FUNCTION_BLOCK FB_IEDServerSession IMPLEMENTS I_ScsmAbortIndEventSink, I_ScsmAssociateIndEventSink, I_ScsmReleaseIndEventSink
VAR_INPUT
	fbConnection		: FB_iec61850ConnectionClass := (ipAbortInd:=THIS^, ipAssociateInd:=THIS^, ipReleaseInd:=THIS^);
END_VAR
VAR
	_bAbort				: BOOL; (* Rising edge activates AbortReq() command execution *)
	_bDisconnect		: BOOL; (* Rising edge activates ReleaseReq() command execution *)
	
	state				: BYTE;
	eState				: E_AsyncEnvironmentState; (* Environment state *)
	bBusy				: BOOL; (* If TRUE => command execution is busy *)
	bSuccess			: BOOL;
	ipResult			: I_AsyncServiceResultClass;
	sLastErrorResult	: T_MaxString;
	fbAbortReason		: FB_ServiceErrorClass := (stError:=SUCCESS_EVENT);
	sLastAbortReason	: T_MaxString;
END_VAR

fbConnection.Execute();
eState:= fbConnection.eState;

(* Execute server control block implementations *)
fbIED.IEDLD1.LLN0.urcb101.Server.Execute();
fbIED.IEDLD1.LLN0.brcb101.Server.Execute();

{region Controlmodel}
fbIED.IEDLD1.ATCC1.BndCtrChg.fbControl.Execute();
fbIED.IEDLD1.ATCC1.TapChg.fbControl.Execute();
fbIED.IEDLD1.ATCC1.TapPos.fbControl.Execute();

fbIED.IEDLD1.CSWI1.Pos.fbControl.Execute();

fbIED.IEDLD1.LEDGGIO1.AnOut1.fbControl.Execute();
fbIED.IEDLD1.LEDGGIO1.DPCSO1.fbControl.Execute();
fbIED.IEDLD1.LEDGGIO1.ISCSO1.fbControl.Execute();
fbIED.IEDLD1.LEDGGIO1.SPCSO1.fbControl.Execute();

fbIED.IEDLD1.LEDGGIO2.AnOut1.fbControl.Execute();
fbIED.IEDLD1.LEDGGIO2.DPCSO1.fbControl.Execute();
fbIED.IEDLD1.LEDGGIO2.ISCSO1.fbControl.Execute();
fbIED.IEDLD1.LEDGGIO2.SPCSO1.fbControl.Execute();

fbIED.IEDLD1.LEDGGIO3.AnOut1.fbControl.Execute();
fbIED.IEDLD1.LEDGGIO3.DPCSO1.fbControl.Execute();
fbIED.IEDLD1.LEDGGIO3.ISCSO1.fbControl.Execute();
fbIED.IEDLD1.LEDGGIO3.SPCSO1.fbControl.Execute();

fbIED.IEDLD1.LEDGGIO4.AnOut1.fbControl.Execute();
fbIED.IEDLD1.LEDGGIO4.DPCSO1.fbControl.Execute();
fbIED.IEDLD1.LEDGGIO4.ISCSO1.fbControl.Execute();
fbIED.IEDLD1.LEDGGIO4.SPCSO1.fbControl.Execute();

fbIED.IEDLD1.LEDGGIO5.AnOut1.fbControl.Execute();
fbIED.IEDLD1.LEDGGIO5.DPCSO1.fbControl.Execute();
fbIED.IEDLD1.LEDGGIO5.ISCSO1.fbControl.Execute();
fbIED.IEDLD1.LEDGGIO5.SPCSO1.fbControl.Execute();

fbIED.IEDLD1.LEDGGIO6.AnOut1.fbControl.Execute();
fbIED.IEDLD1.LEDGGIO6.DPCSO1.fbControl.Execute();
fbIED.IEDLD1.LEDGGIO6.ISCSO1.fbControl.Execute();
fbIED.IEDLD1.LEDGGIO6.SPCSO1.fbControl.Execute();

fbIED.IEDLD1.LEDGGIO7.AnOut1.fbControl.Execute();
fbIED.IEDLD1.LEDGGIO7.DPCSO1.fbControl.Execute();
fbIED.IEDLD1.LEDGGIO7.ISCSO1.fbControl.Execute();
fbIED.IEDLD1.LEDGGIO7.SPCSO1.fbControl.Execute();

fbIED.IEDLD1.LEDGGIO8.AnOut1.fbControl.Execute();
fbIED.IEDLD1.LEDGGIO8.DPCSO1.fbControl.Execute();
fbIED.IEDLD1.LEDGGIO8.ISCSO1.fbControl.Execute();
fbIED.IEDLD1.LEDGGIO8.SPCSO1.fbControl.Execute();

fbIED.IEDLD1.XCBR1.Pos.fbControl.Execute();

fbIED.IEDLD1.LLN0.Mod_.fbControl.Execute();
{endregion}

CASE state OF
	0: (* Initial state *)
		IF _bAbort THEN (* Abort connection => execute AbortReq() command *)
			_bAbort:= FALSE;
			bSuccess:= fbConnection.AbortReq(ipReason:=fbAbortReason, ipSink:=0, ipResult=>ipResult);
			state:= SEL(bSuccess, 100, 1);
		ELSIF eState = E_AsyncEnvironmentState.Established AND _bDisconnect THEN (* Close/release connection => execute ReleaseReq() command *)
			_bDisconnect:= FALSE;
			bSuccess:= fbConnection.ReleaseReq(ipSink:=0, ipResult=>ipResult);
			state:= SEL(bSuccess, 100, 1);
		ELSIF eState = E_AsyncEnvironmentState.Established THEN (* Connection established => exchange IED data *)
			state:= 10;
		END_IF
		_bDisconnect:= FALSE;
		(*==================================================================================================================================================================*)
	1: (* Wait for AbortReq() or ReleaseReq() command completion *)
		IF ipResult <> 0 THEN
			ipResult.Execute();
			IF NOT (bBusy:=ipResult.IsBusy()) THEN
				state:= SEL(ipResult.IsCompleted(), 100(* failed or aborted *), 0(* succeeded *));
			END_IF
		END_IF
		(*==================================================================================================================================================================*)
	10: (* connection established *)
		state:= 0;
		(*==================================================================================================================================================================*)
	100: (* Error state *)
		state:= 0;
		IF ipResult <> 0 THEN
			sLastErrorResult:= ipResult.Dump();
		END_IF
END_CASE

PROPERTY bAbort : BOOL
SET
_bAbort:= bAbort;
END_SET
END_PROPERTY

PROPERTY bDisconnect : BOOL
SET
_bDisconnect:= bDisconnect;
END_SET
END_PROPERTY

(* This method receives IEC61850::Abort.ind primitive. *)
METHOD OnAbortInd
VAR_INPUT
	ipAA		: I_ScsmAssociationClass; (* Application association. If = 0 => optional. *)
	bPAbort		: BOOL; (* TRUE => P-Abort.request(), issued by provider, FALSE => Abort.request(), issued by user. *)
	ipReason	: I_ServiceErrorClass; (* Abort reason. *)
	ipData		: I_BaseStreamClass; (* Optional data. If = 0 => default, no data. *)
END_VAR
VAR
END_VAR
IF ipReason <> 0 THEN
	sLastAbortReason:= ipReason.Dump();
END_IF
END_METHOD

(* This method receives IEC61850::Associate.ind primitive. *)
METHOD OnAssociateInd : BOOL
VAR_INPUT
	ipAA	: I_ScsmAssociationClass; (* Application association. If = 0 => optional. *)
END_VAR
VAR_OUTPUT
	ipResult : I_AsyncServiceResultClass;
END_VAR
VAR
END_VAR
sLastAbortReason:= '';
sLastErrorResult:= '';
OnAssociateInd:= fbConnection.AssociateRsp(ipResult=>ipResult);
END_METHOD

(* This method receives IEC61850::Release.ind primitive. *)
METHOD OnReleaseInd : BOOL
VAR_INPUT
	ipAA	: I_ScsmAssociationClass; (* Application association. If = 0 => optional. *)
END_VAR
VAR_OUTPUT
	ipResult: I_AsyncServiceResultClass;
END_VAR
VAR
END_VAR
OnReleaseInd:= fbConnection.ReleaseRsp(ipResult=>ipResult);
END_METHOD

END_FUNCTION_BLOCK
